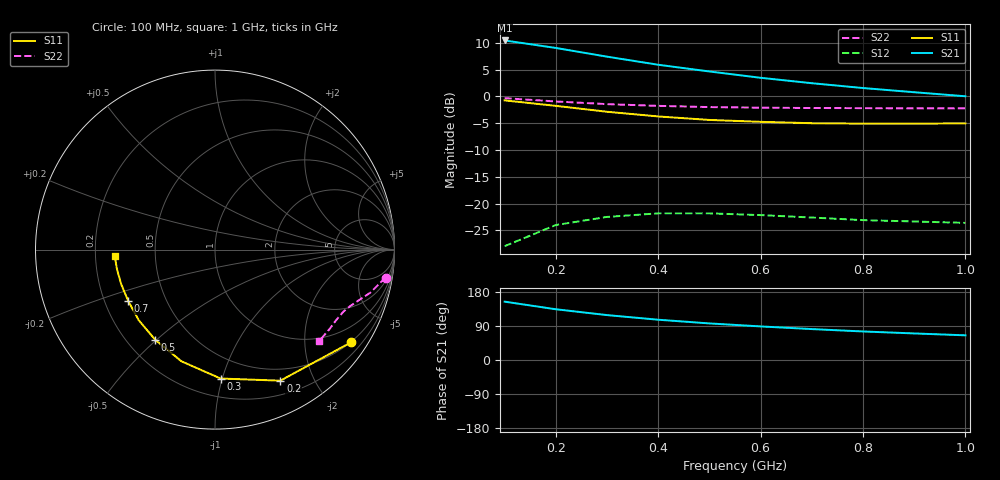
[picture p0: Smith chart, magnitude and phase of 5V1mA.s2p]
#  HZ  S  MA  R  50.0000
! Device:15GN03CA
! "! Bias:VCE=5V, IC=1mA  "
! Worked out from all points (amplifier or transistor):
!   10 points, 100 MHz to 1 GHz, reference 50 ohm
!   highest |S21| = 10.4 dB at 100 MHz (marker M1)
!   |S21| within 3 dB of that: start of sweep to 298.4 MHz
!   unconditionally stable (mu >= 1): 581.6 MHz to end of sweep
!   at 200 MHz: K = 0.36, MSG = 16.5 dB, |S12| = -24.0 dB
!   at 600 MHz: K = 1.04, MAG = 11.6 dB, |S12| = -22.2 dB
!   at 1 GHz: K = 1.73, MAG = 6.8 dB, |S12| = -23.6 dB
!   S11 on the Smith chart (normalised r, x): 100 MHz: 0.49, -3.18; 200 MHz: 0.36, -1.56; 300 MHz: 0.33, -0.99; 500 MHz: 0.31, -0.50; 700 MHz: 0.30, -0.25; 1 GHz: 0.28, -0.03
1e8  0.918 -34.2  3.328 154.0  0.04 67.1  0.963 -9.3
2e8  0.816 -63.5  2.833 133.9  0.063 50.5  0.897 -15.6
3e8  0.719 -87.5  2.349 118.5  0.075 39.9  0.847 -19.6
4e8  0.65 -106.7  1.974 106.3  0.081 33.7  0.816 -22.7
5e8  0.603 -123.5  1.709 96.5  0.081 30.4  0.795 -25.7
6e8  0.579 -137.2  1.492 88.6  0.078 30.5  0.785 -28.6
7e8  0.562 -149.3  1.328 81.6  0.074 30.6  0.779 -31.4
8e8  0.557 -159.6  1.197 75.3  0.07 35.0  0.777 -34.7
9e8  0.557 -168.6  1.094 70.1  0.068 41.6  0.773 -38.0
1e9  0.56 -176.4  1.003 65.1  0.066 50.3  0.773 -41.2
